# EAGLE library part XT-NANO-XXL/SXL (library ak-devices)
AK-NORD XT-NANO-XXL/SXL
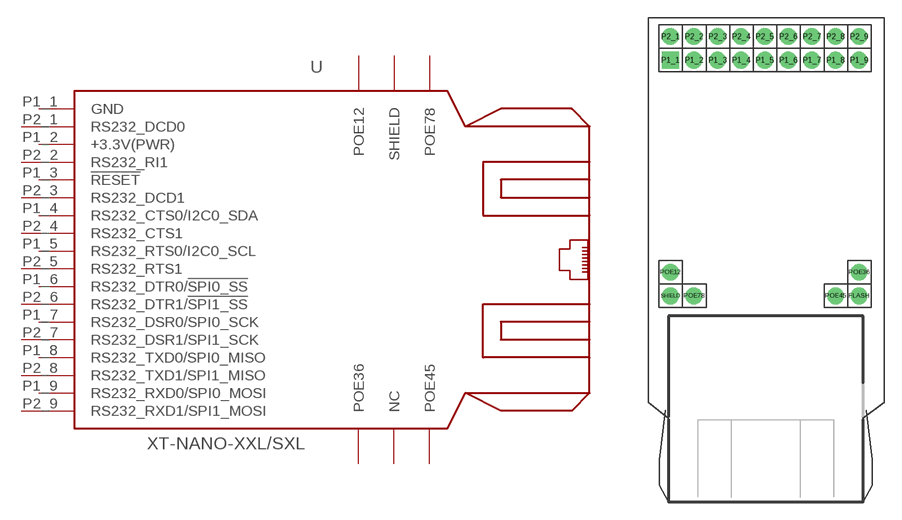
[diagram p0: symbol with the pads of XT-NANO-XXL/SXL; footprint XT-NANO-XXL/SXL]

Designator prefix -

## XT-NANO-XXL/SXL  [XT-NANO-XXL/SXL]
FLASH  NC  nc
P1_1  GND  pas
P1_2  +3.3V(PWR)  pas
P1_3  !RESET  in
P1_4  RS232_CTS0/I2C0_SDA  pas
P1_5  RS232_RTS0/I2C0_SCL  pas
P1_6  RS232_DTR0/!SPI0_SS!  pas
P1_7  RS232_DSR0/SPI0_SCK  pas
P1_8  RS232_TXD0/SPI0_MISO  pas
P1_9  RS232_RXD0/SPI0_MOSI  pas
P2_1  RS232_DCD0  pas
P2_2  RS232_RI1  pas
P2_3  RS232_DCD1  pas
P2_4  RS232_CTS1  pas
P2_5  RS232_RTS1  pas
P2_6  RS232_DTR1/!SPI1_SS!  pas
P2_7  RS232_DSR1/SPI1_SCK  pas
P2_8  RS232_TXD1/SPI1_MISO  pas
P2_9  RS232_RXD1/SPI1_MOSI  pas
POE12  POE12  pas
POE36  POE36  pas
POE45  POE45  pas
POE78  POE78  pas
SHIELD  SHIELD  pas

## Footprint XT-NANO-XXL/SXL (pad centres in mm)
AK-NORD XT-NANO-XXL/SXL
drill 0.813 pad 1.422: FLASH 8,-10; P1_2 -6,10; P1_3 -4,10; P1_4 -2,10; P1_5 0,10; P1_6 2,10; P1_7 4,10; P1_8 6,10; P1_9 8,10; P2_1 -8,12; P2_2 -6,12; P2_3 -4,12; P2_4 -2,12; P2_5 0,12; P2_6 2,12; P2_7 4,12; P2_8 6,12; P2_9 8,12; POE12 -8,-8; POE36 8,-8; POE45 6,-10; POE78 -6,-10; SHIELD -8,-10
drill 0.813 pad 1.422 square: P1_1 -8,10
